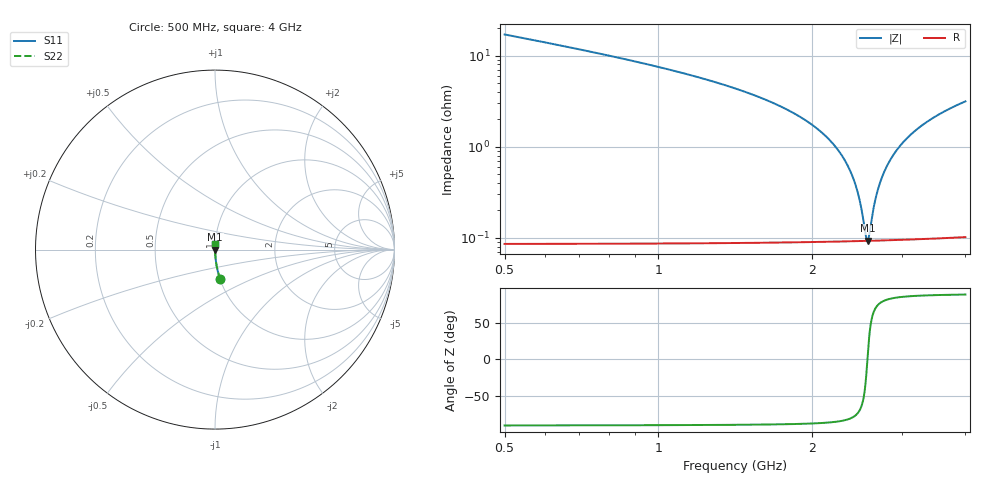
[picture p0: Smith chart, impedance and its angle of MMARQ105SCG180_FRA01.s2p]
! MMARQ105SCG180_FRA01  S-PARAMETER MODEL  ( General Type )
! Model Generated by TAIYO YUDEN Corporation (http://www.ty-top.com)
! Version 1.0
! TAIYO YUDEN Control No. 200326
! Copyright(c) 2020 TAIYO YUDEN CO.,LTD. All Rights Reserved.
! Product Description (link to TY-COMPAS)
! https://ds.yuden.co.jp/TYCOMPAS/or/detail?pn=MMARQ105SCG180JFRA01&u=M
! Products Name : Multilayer Ceramic Capacitors
! Characteristics :
!  Capacitance : 18 pF , Rated Voltage : 250V , TCC : CG / C0G
!  Case Size : 1.0 x 0.5 / 0.039 x 0.02 [mm/inch] , Thickness : 0.5 / 0.02 [mm/inch]
!  (Conditions: Temperature = 25 degC , DC Bias Current/Voltage = 0A / 0V)
! External Node Assignments :
!  1  o---| |---o  2
! GND o---------o GND
! Frequency Range : 500MHz  -  4GHz  [ 401 STEP ]
# MHz S RI R 50
! Freq[MHz].  S11 Real  S11 Imag  S21 Real  S21 Imag  S12 Real  S12 Imag  S22 Real  S22 Imag
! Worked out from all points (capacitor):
!   401 points, 500 MHz to 4 GHz, reference 50 ohm
!   read as one part in series: C = 18 pF near 517.5 MHz
!   lowest |Z| = 93 mohm at 2.574 GHz (marker M1)
!   series resonance near 2.571 GHz, so ESL is about 210 pH
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500  0.029 -0.1652  0.971 0.1652  0.971 0.1652  0.029 -0.1652
753.75  0.0122 -0.1059  0.9878 0.1059  0.9878 0.1059  0.0122 -0.1059
1086.25  0.00531 -0.0665  0.9947 0.0665  0.9947 0.0665  0.00531 -0.0665
1672.5  0.00181 -0.0304  0.9982 0.0304  0.9982 0.0304  0.00181 -0.0304
2013.75  0.00119 -0.0169  0.9988 0.0169  0.9988 0.0169  0.00119 -0.0169
2145  0.00106 -0.0125  0.9989 0.0125  0.9989 0.0125  0.00106 -0.0125
2250  0.000994 -0.00918  0.999 0.00918  0.999 0.00918  0.000994 -0.00918
2346.25  0.000954 -0.00628  0.999 0.00628  0.999 0.00628  0.000954 -0.00628
2425  0.000934 -0.00401  0.9991 0.00401  0.9991 0.00401  0.000934 -0.00401
2486.25  0.000927 -0.0023  0.9991 0.0023  0.9991 0.0023  0.000927 -0.0023
2556.25  0.000925 -0.000388  0.9991 0.000388  0.9991 0.000388  0.000925 -0.000388
2573.75  0.000926 8.04e-05  0.9991 -8.04e-05  0.9991 -8.04e-05  0.000926 8.04e-05
2591.25  0.000927 0.000546  0.9991 -0.000546  0.9991 -0.000546  0.000927 0.000546
2652.5  0.000935 0.00215  0.9991 -0.00215  0.9991 -0.00215  0.000935 0.00215
2696.25  0.000943 0.00327  0.9991 -0.00327  0.9991 -0.00327  0.000943 0.00327
2757.5  0.000959 0.00482  0.999 -0.00482  0.999 -0.00482  0.000959 0.00482
2836.25  0.000986 0.00676  0.999 -0.00676  0.999 -0.00676  0.000986 0.00676
2941.25  0.00103 0.00927  0.999 -0.00927  0.999 -0.00927  0.00103 0.00927
3072.5  0.00111 0.0123  0.9989 -0.0123  0.9989 -0.0123  0.00111 0.0123
3230  0.00121 0.0158  0.9988 -0.0158  0.9988 -0.0158  0.00121 0.0158
3422.5  0.00137 0.0199  0.9986 -0.0199  0.9986 -0.0199  0.00137 0.0199
4000  0.002 0.0313  0.998 -0.0313  0.998 -0.0313  0.002 0.0313
